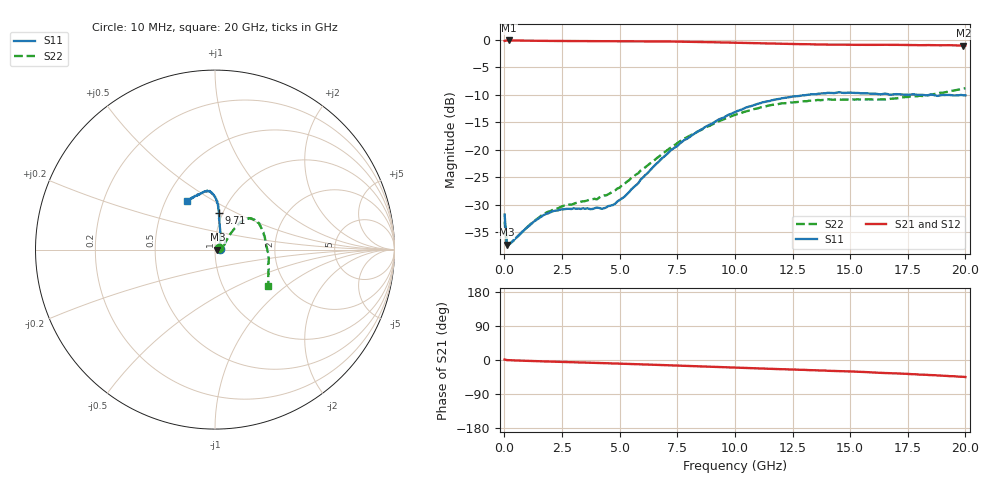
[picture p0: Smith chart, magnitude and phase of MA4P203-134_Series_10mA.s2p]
! AWR Design Environment (9226) Thu Aug 19 14:29:25 2021
! Document = '10mA'
! nPorts: 2, nXvals: 201
# GHz S DB R 50
!Freq DBS11 AngS11 DBS21 AngS21 DBS12 AngS12 DBS22 AngS22
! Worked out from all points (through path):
!   201 points, 10 MHz to 20 GHz, reference 50 ohm
!   highest |S21| = -0.17 dB at 210 MHz (marker M1); lowest = -1.1 dB at 19.91 GHz (marker M2)
!   group delay of S21, straight-line fit = 5.95 ps
!   lowest |S11| = -37.3 dB at 110 MHz (marker M3), VSWR 1.03, Z = 51.4 - j0.0268 ohm
!   |S11| at or under -10 dB: start of sweep to 13.21 GHz; 17.85 GHz to 18.5 GHz (653.6 MHz wide, 3.6 % of centre); 18.52 GHz to end of sweep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
!   |S22| runs from -37.5 to -8.9 dB; largest |S21 - S12| = 0.043
!   S11 on the Smith chart (normalised r, x): 10 MHz: 1.05, +0.01; 9.71 GHz: 0.96, +0.41; 20 GHz: 0.64, +0.38
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0.01  -31.78 6.1  -0.25 1.3  -0.23 0.9  -33.06 21.2
0.11  -37.27 -1.1  -0.17 -0.2  -0.16 -0.2  -37.53 -1.6
0.21  -37.17 1.4  -0.17 -0.5  -0.16 -0.5  -37.20 3.0
1.21  -33.31 -4.2  -0.22 -2.7  -0.21 -2.6  -33.24 -3.8
1.71  -31.87 -11.1  -0.25 -3.6  -0.23 -3.4  -31.71 -10.8
2.41  -30.90 -17.2  -0.27 -4.8  -0.26 -4.5  -30.47 -16.3
3.41  -30.66 -11.7  -0.28 -6.7  -0.26 -6.1  -29.38 -11.7
4.01  -30.50 -0.0  -0.29 -7.8  -0.27 -7.2  -29.03 -2.8
4.21  -30.74 7.6  -0.29 -8.1  -0.27 -7.5  -28.44 0.2
4.71  -30.06 22.3  -0.30 -9.0  -0.28 -8.4  -27.54 8.9
5.21  -28.55 39.2  -0.31 -10.0  -0.28 -9.3  -26.27 18.4
6.71  -22.14 67.6  -0.34 -13.1  -0.32 -12.3  -21.25 40.0
7.81  -18.23 77.0  -0.40 -15.5  -0.39 -14.5  -17.99 45.5
9.71  -13.70 84.2  -0.55 -19.6  -0.54 -18.3  -14.15 47.2
10.01  -13.16 84.3  -0.58 -20.3  -0.57 -18.9  -13.68 47.3
11.21  -11.40 87.2  -0.70 -22.8  -0.69 -21.1  -12.26 44.6
13.41  -9.95 93.9  -0.88 -26.8  -0.84 -25.2  -11.06 34.6
14.51  -9.57 97.5  -0.95 -29.3  -0.88 -27.3  -10.87 27.5
16.71  -10.01 108.2  -0.97 -34.8  -0.89 -32.4  -10.79 2.9
18.21  -10.08 116.4  -1.02 -38.7  -0.92 -37.1  -10.25 -15.8
19.91  -10.14 120.9  -1.10 -44.3  -1.02 -43.1  -8.93 -33.7
20  -10.14 119.7  -1.09 -45.0  -1.03 -43.3  -8.86 -34.6
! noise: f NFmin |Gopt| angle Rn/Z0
0.01  0  1  0  2e-20
2.21  0  1  0  2e-20
4.41  0  1  0  2e-20
6.61  0  1  0  2e-20
8.81  0  1  0  2e-20
11.11  0  1  0  2e-20
13.31  0  1  0  2e-20
15.51  0  1  0  2e-20
17.71  0  1  0  2e-20
20  0  1  0  2e-20
